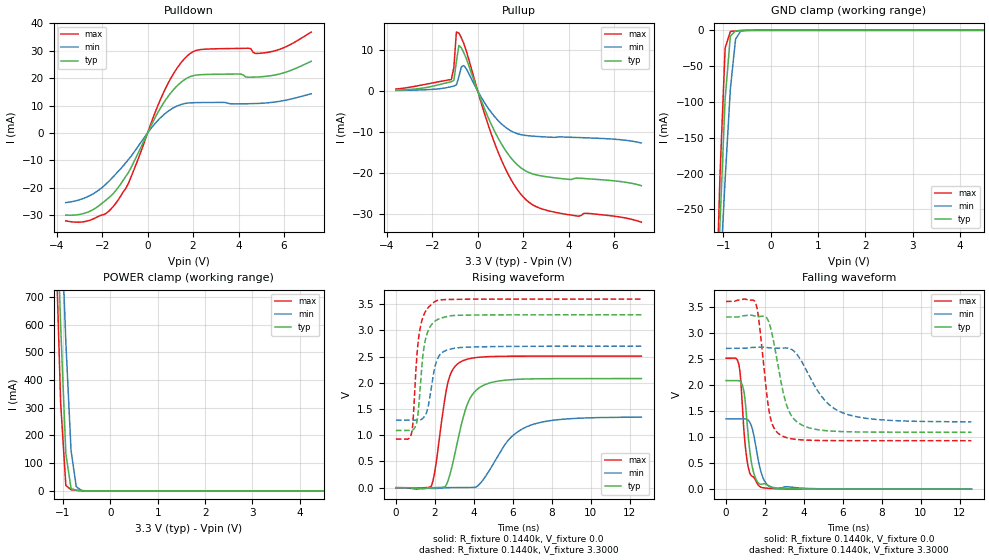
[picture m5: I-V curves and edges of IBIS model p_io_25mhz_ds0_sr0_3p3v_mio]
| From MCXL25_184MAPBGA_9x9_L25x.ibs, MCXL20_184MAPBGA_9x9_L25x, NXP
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[Model] p_io_25mhz_ds0_sr0_3p3v_mio
|   Model p_io_25mhz_ds0_sr0_3p3v_mio
| This model was characterised for following simulation conditions:
| External (pad) voltage:
|   - Typ: 3.3V,   - Min: 2.7V,   - Max: 3.6V
| Library cells for typ/min/max conditions are connected as defined below:
|  pad - External Pad
|  ipp_do_lv - Core Input
|  ipp_obe_lv - Output Buffer Enable
|  IOGC - NC
|  REFH3V3 - REFH3V3
|  REFL3V3 - REFL3V3
|  ZI - NC
|  abut_ncal_vddio[1] - vddio
|  abut_ncal_vddio[2] - vddio
|  abut_ncal_vddio[3] - vssio
|  abut_ncal_vddio[4] - vddio
|  abut_ncal_vddio[5] - vddio
|  abut_ncal_vddio[6] - vssio
|  abut_pcal_vddio[1] - vssio
|  abut_pcal_vddio[2] - vssio
|  abut_pcal_vddio[3] - vddio
|  abut_pcal_vddio[4] - vssio
|  abut_pcal_vddio[5] - vssio
|  abut_pcal_vddio[6] - vddio
|  ipp_do_1p8v - ipp_do_1p8v
|  ipp_dse_lv - 0
|  ipp_eftd_lv - NC
|  ipp_ina_mux_vddio - NC
|  ipp_ina_mux_vddio[0] - NC
|  ipp_ina_mux_vddio[1] - NC
|  ipp_ina_r0_vddio - NC
|  ipp_ina_r0a_vddio - NC
|  ipp_ina_r0b_vddio - NC
|  ipp_ina_r0c_vddio - NC
|  ipp_ina_r0d_vddio - NC
|  ipp_ina_r0e_vddio - NC
|  ipp_ina_r0f_vddio - NC
|  ipp_ina_r300_vddio - NC
|  ipp_ina_r300a_vddio - NC
|  ipp_ina_r300b_vddio - NC
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Model_type I/O
Polarity   Non-Inverting
Enable   Active-High
Vinl =   0.9900V
Vinh =   2.3100V
Vmeas =  1.6500V
Cref =   30.0000pF
Rref =   1.0000M
Vref =   3.3000V
C_comp   1.2813pF   1.2310pF   1.3501pF
|C_comp_pullup   0.5366pF   0.5680pF   0.5152pF
|C_comp_pulldown   0.6537pF   0.6898pF   0.6249pF
[Model Spec]
| variable   typ   min   max
Vinh   2.3100V   1.8900V   2.5200V
Vinl   0.9900V   0.8100V   1.0800V
[Temperature Range]   25.0000   0.1250k   -40.0000
[Voltage Range]   3.3000V   2.7000V   3.6000V
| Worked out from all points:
|   slope of the pulldown table from 0 to 0.495 V, typ, clamps not added: 61.2 ohm
|   slope of the pullup table from 0 to 0.495 V, typ, clamps not added: 71.6 ohm
|   GND clamp passes 1 mA (typ) near -0.74 V on its own axis
|   POWER clamp passes 1 mA (typ) near -0.62 V on its own axis
|   rising waveform, R_fixture 0.1440k, V_fixture 0.0: 20-80 % time 865ps typ, 1.6ns min, 593ps max; typ from 0 V to 2.08 V
|   rising waveform, R_fixture 0.1440k, V_fixture 3.3000: 20-80 % time 369ps typ, 425ps min, 343ps max; typ from 1.09 V to 3.3 V
|   falling waveform, R_fixture 0.1440k, V_fixture 0.0: 20-80 % time 363ps typ, 446ps min, 330ps max; typ from 2.08 V to 0 V
|   falling waveform, R_fixture 0.1440k, V_fixture 3.3000: 20-80 % time 757ps typ, 1.53ns min, 485ps max; typ from 3.3 V to 1.09 V
[Pulldown]
|Voltage   I(typ)   I(min)   I(max)
-3.6V     -30mA      -25.44mA   -32.1mA
-2.5V     -28.44mA   -22.71mA   -31.77mA
-1.84V    -24.58mA   -18.74mA   -29.46mA
-1.4V     -21.04mA   -15mA      -25.71mA
-850mV    -14.54mA   -9.776mA   -18.5mA
800mV     12.14mA    7.262mA    16.45mA
1.35V     17.61mA    10.02mA    24.31mA
1.9V      20.65mA    10.99mA    29.16mA
4.43V     20.35mA    10.67mA    30.93mA
4.76V     20.4mA     10.74mA    29.02mA
5.31V     20.76mA    11.02mA    29.46mA
7.2V      26.15mA    14.29mA    36.82mA
[Pullup]
|Voltage   I(typ)   I(min)   I(max)
-3.6V     251.1uA    138.4uA    485.2uA
-1.16V    2.273mA    1.07mA     2.803mA
-1.05V    2.605mA    1.214mA    5.78mA
-940mV    7.098mA    1.466mA    14.39mA
-830mV    11.13mA    3.483mA    14.16mA
-720mV    10.55mA    5.906mA    12.99mA
-610mV    9.34mA     6.201mA    11.54mA
820mV     -10.68mA   -6.751mA   -13.85mA
1.48V     -16.44mA   -9.786mA   -21.76mA
2.03V     -19.26mA   -10.79mA   -26.03mA
3.35V     -21.17mA   -11.31mA   -29.54mA
7.2V      -23.11mA   -12.69mA   -32.03mA
[GND_clamp]
|Voltage   I(typ)   I(min)   I(max)
-3.6V     -5.285A    -4.099A    -6.854A
-1.18V    -466mA     -495.3mA   -458.9mA
-1.07V    -271.1mA   -348.5mA   -204.6mA
-960mV    -95.66mA   -207.9mA   -24.82mA
-850mV    -8.126mA   -81.84mA   -1.536mA
-740mV    -740.4uA   -12.14mA   -755uA
-630mV    -283.6uA   -928.1uA   -319.7uA
-300mV    -497.8nA   -2.865uA   -109.5nA
7.2V      0A         0A         0A
[POWER_clamp]
|Voltage   I(typ)   I(min)   I(max)
-3.6V     14.48A     12.95A     16.35A
-1.16V    1.177A     1.535A     951.2mA
-1.05V    598.3mA    1.032A     318mA
-940mV    134.2mA    537.3mA    19.98mA
-830mV    8.694mA    145.4mA    4.231mA
-720mV    2.123mA    15.37mA    2.22mA
-610mV    848.6uA    1.85mA     839.5uA
7.2V      0A         0A         0A
[Ramp]
| variable   typ   min   max
dV/dt_r  1.2495/0.8651n   0.8077/1.6035n   1.5064/0.5933n
dV/dt_f  1.3251/0.7572n   0.8455/1.5282n   1.6027/0.4851n
R_load = 0.1440k
[Rising Waveform]
R_fixture= 0.1440k
V_fixture= 0.0
V_fixture_min= 0.0
V_fixture_max= 0.0
|time   V(typ)   V(min)   V(max)
0s        4.67nV     159.2nV    15.81nV
1.811ns   103.5uV    -14.27mV   28.53mV
2.023ns   2.341mV    -15.6mV    366.7mV
2.65ns    108.9mV    902.7uV    1.978V
3.33ns    1.163V     1.642mV    2.404V
3.904ns   1.766V     3.622mV    2.472V
4.866ns   2.005V     371mV      2.503V
5.871ns   2.06V      949mV      2.509V
7.012ns   2.077V     1.204V     2.51V
12.6ns    2.083V     1.346V     2.511V
[Rising Waveform]
R_fixture= 0.1440k
V_fixture= 3.3000
V_fixture_min= 2.7000
V_fixture_max= 3.6000
|time   V(typ)   V(min)   V(max)
0s        1.091V     1.289V     928.9mV
788.1ps   1.091V     1.289V     1.019V
881.2ps   1.107V     1.289V     1.286V
1.023ns   1.19V      1.289V     2.234V
1.203ns   1.7V       1.29V      2.956V
1.477ns   2.759V     1.365V     3.336V
2.016ns   3.181V     2.325V     3.556V
2.39ns    3.245V     2.584V     3.587V
3.294ns   3.292V     2.675V     3.596V
12.6ns    3.3V       2.7V       3.6V
[Falling Waveform]
R_fixture= 0.1440k
V_fixture= 0.0
V_fixture_min= 0.0
V_fixture_max= 0.0
|time   V(typ)   V(min)   V(max)
0s        2.083V     1.348V     2.511V
620.7ps   2.084V     1.348V     2.438V
728.4ps   2.07V      1.348V     2.204V
841.2ps   1.991V     1.348V     1.57V
982.1ps   1.689V     1.349V     844.5mV
1.157ns   945.2mV    1.315V     393.4mV
1.407ns   329.5mV    1.064V     231.3mV
1.767ns   92.82mV    366.8mV    41.64mV
2.572ns   23.71mV    16.14mV    8.637mV
12.6ns    234.6nV    16.61uV    19.32nV
[Falling Waveform]
R_fixture= 0.1440k
V_fixture= 3.3000
V_fixture_min= 2.7000
V_fixture_max= 3.6000
|time   V(typ)   V(min)   V(max)
0s        3.3V       2.7V       3.6V
1.511ns   3.319V     2.721V     3.579V
1.695ns   3.312V     2.725V     3.208V
2.244ns   3.151V     2.709V     1.426V
2.815ns   2.071V     2.707V     1.034V
3.155ns   1.563V     2.704V     982.6mV
3.604ns   1.301V     2.602V     953.7mV
4.915ns   1.13V      1.775V     933mV
5.944ns   1.104V     1.471V     930.2mV
12.6ns    1.091V     1.291V     928.9mV
